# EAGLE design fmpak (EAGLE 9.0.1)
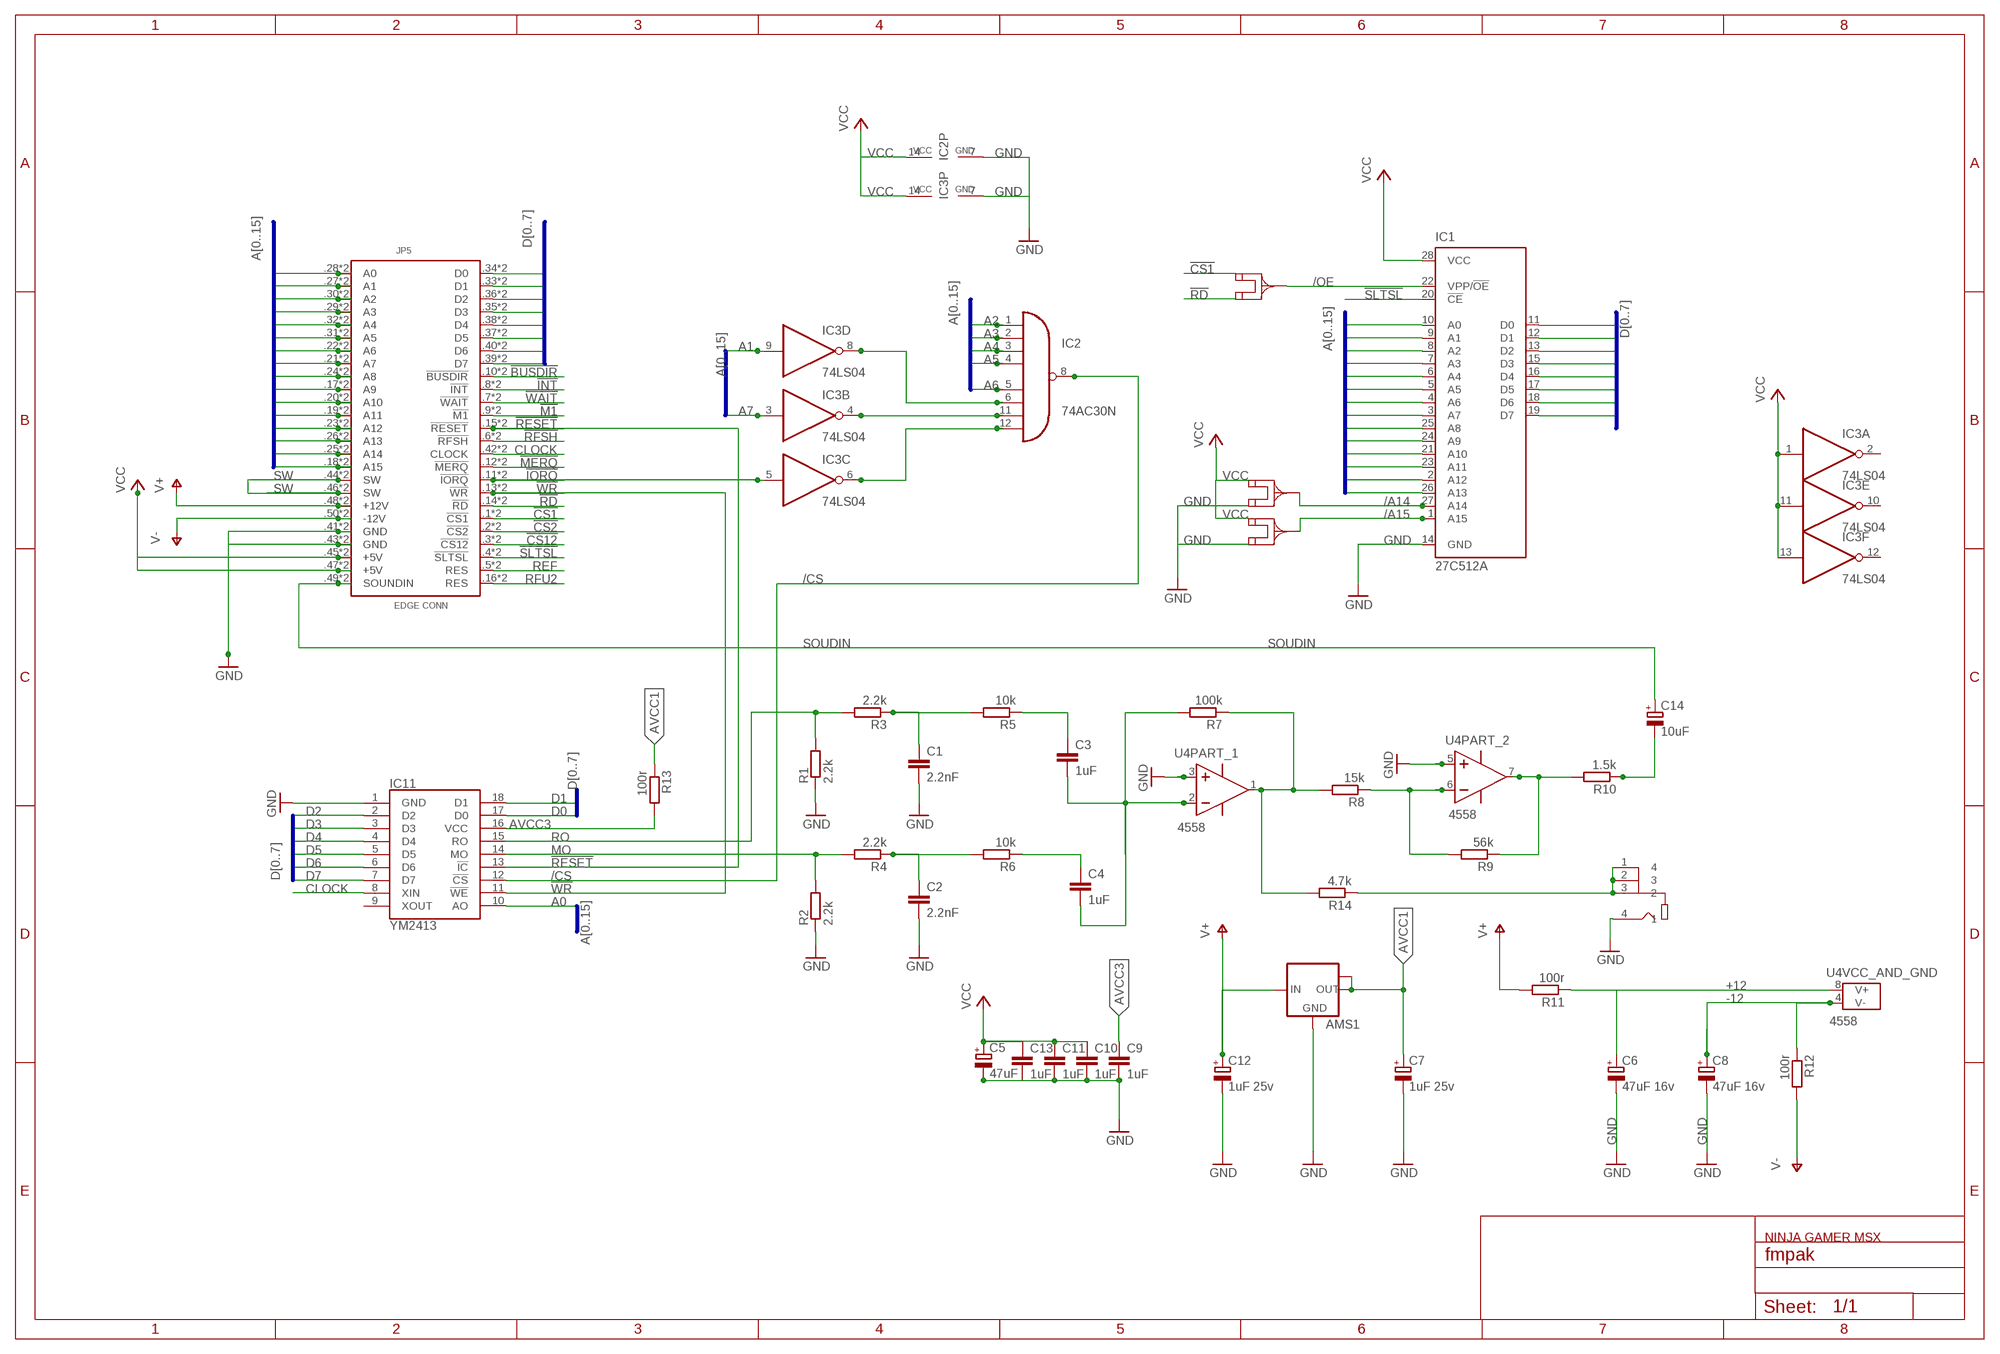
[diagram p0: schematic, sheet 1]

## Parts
AMS1  LM1117IMPX-5.0  [SOT223]
C1  2.2nF  C-EUC0805  [C0805]
C2  2.2nF  C-EUC0805  [C0805]
C3  1uF  C-EUC0805  [C0805]
C4  1uF  C-EUC0805  [C0805]
C5  47uF  CPOL-EUSMCC  [SMC_C]
C6  47uF 16v  CPOL-EUSMCC  [SMC_C]
C7  1uF 25v  CPOL-EUSMCB  [SMC_B]
C8  47uF 16v  CPOL-EUSMCC  [SMC_C]
C9  1uF  C-EUC0805  [C0805]
C10  1uF  C-EUC0805  [C0805]
C11  1uF  C-EUC0805  [C0805]
C12  1uF 25v  CPOL-EUSMCB  [SMC_B]
C13  1uF  C-EUC0805  [C0805]
C14  10uF  CPOL-EUSMCB  [SMC_B]
IC1  27C512A  27C512AP  [DIL28-6]
IC2  74AC30N  [DIL14]
IC3  74LS04  74LS04D  [SO14]
IC11  YM2413  [DIP762W56P254L2300H450Q18N]
J1  RCJ-04X  [CUI_RCJ-041]
JP5  MSXCART1  [MSXCART]
R1  2.2k  R-EU_R0805  [R0805]
R2  2.2k  R-EU_R0805  [R0805]
R3  2.2k  R-EU_R0805  [R0805]
R4  2.2k  R-EU_R0805  [R0805]
R5  10k  R-EU_R0805  [R0805]
R6  10k  R-EU_R0805  [R0805]
R7  100k  R-EU_R0805  [R0805]
R8  15k  R-EU_R0805  [R0805]
R9  56k  R-EU_R0805  [R0805]
R10  1.5k  R-EU_R0805  [R0805]
R11  100r  R-EU_R0805  [R0805]
R12  100r  R-EU_R0805  [R0805]
R13  100r  R-EU_R0805  [R0805]
R14  4.7k  R-EU_R0805  [R0805]
U4  4558  4558SO8  [SOP8]
U$1  JUMP-SMD  [A0R-JMP]
U$2  JUMP-SMD  [A0R-JMP]
U$3  JUMP-SMD  [A0R-JMP]

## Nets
!BUSDIR: JP5.9(!BUSDIR) JP5..10(!BUSDIR)
!CS1: JP5.1(!CS1) JP5..1(!CS1) U$2.1
!CS2: JP5.2(!CS2) JP5..2(!CS2)
!CS12: JP5.3(!CS12) JP5..3(!CS12)
!INT: JP5.8(!INT) JP5..8(!INT)
!IORQ: IC3.5(C:I) JP5.12(!IORQ) JP5..11(!IORQ)
!M1: JP5.10(!M1) JP5..9(!M1)
!MERQ: JP5.11(!MERQ) JP5..12(!MERQ)
!RD: JP5.14(!RD) JP5..14(!RD) U$2.3
!RESET: IC11.13(!IC) JP5.15(!RESET) JP5..15(!RESET)
!RFSH: JP5.6(!RFSH) JP5..6(!RFSH)
!SLTSL: IC1.20(!CE) JP5.4(!SLTSL) JP5..4(!SLTSL)
!WAIT: JP5.7(!WAIT) JP5..7(!WAIT)
!WR: IC11.11(!WE) JP5.13(!WR) JP5..13(!WR)
+12: C6.+ R11.1 U4.8(VCC_AND_GND:V+)
-12: C8.+ R12.1 U4.4(VCC_AND_GND:V-)
/A14: IC1.27(A14) U$1.2
/A15: IC1.1(A15) U$3.2
/CS: IC2.8(O) IC11.12(!CS)
/OE: IC1.22(VPP/!OE) U$2.2
A0: IC1.10(A0) IC11.10(AO) JP5.28(A0) JP5..28(A0)
A1: IC1.9(A1) IC3.9(D:I) JP5.27(A1) JP5..27(A1)
A2: IC1.8(A2) IC2.1(I0) JP5.30(A2) JP5..30(A2)
A3: IC1.7(A3) IC2.2(I1) JP5.29(A3) JP5..29(A3)
A4: IC1.6(A4) IC2.3(I2) JP5.32(A4) JP5..32(A4)
A5: IC1.5(A5) IC2.4(I3) JP5.31(A5) JP5..31(A5)
A6: IC1.4(A6) IC2.5(I4) JP5.22(A6) JP5..22(A6)
A7: IC1.3(A7) IC3.3(B:I) JP5.21(A7) JP5..21(A7)
A8: IC1.25(A8) JP5.24(A8) JP5..24(A8)
A9: IC1.24(A9) JP5.17(A9) JP5..17(A9)
A10: IC1.21(A10) JP5.20(A10) JP5..20(A10)
A11: IC1.23(A11) JP5.19(A11) JP5..19(A11)
A12: IC1.2(A12) JP5.23(A12) JP5..23(A12)
A13: IC1.26(A13) JP5.26(A13) JP5..26(A13)
A14: JP5.25(A14) JP5..25(A14)
A15: JP5.18(A15) JP5..18(A15)
AVCC1 [vcc]: AMS1.2(OUT) AMS1.TAB(OUT1) C7.+ R13.1
AVCC3: C9.1 IC11.16(VCC) R13.2
CLOCK: IC11.8(XIN) JP5.42(CLOCK) JP5..42(CLOCK)
D0: IC1.11(D0) IC11.17(D0) JP5.34(D0) JP5..34(D0)
D1: IC1.12(D1) IC11.18(D1) JP5.33(D1) JP5..33(D1)
D2: IC1.13(D2) IC11.2(D2) JP5.36(D2) JP5..36(D2)
D3: IC1.15(D3) IC11.3(D3) JP5.35(D3) JP5..35(D3)
D4: IC1.16(D4) IC11.4(D4) JP5.38(D4) JP5..38(D4)
D5: IC1.17(D5) IC11.5(D5) JP5.37(D5) JP5..37(D5)
D6: IC1.18(D6) IC11.6(D6) JP5.40(D6) JP5..40(D6)
D7: IC1.19(D7) IC11.7(D7) JP5.39(D7) JP5..39(D7)
GND: AMS1.1(GND) C1.2 C2.2 C5.- C6.- C7.- C8.- C9.2 C10.2 C11.2 C12.- C13.2 IC1.14(GND) IC2.7(GND) IC3.7(P:GND) IC11.1(GND) J1.4 JP5.41(GND) JP5.43(GND) JP5..41(GND) JP5..43(GND) R1.1 R2.1 U4.3(PART_1:IN+) U4.5(PART_2:IN+) U$1.3 U$3.3
MO: IC11.14(MO) R2.2 R4.2
N$2: C1.1 R3.1 R5.2
N$3: C3.1 R5.1
N$5: C2.1 R4.1 R6.2
N$6: C4.1 R6.1
N$7: C3.2 C4.2 R7.2 U4.2(PART_1:IN-)
N$8: R7.1 R8.2 R14.2 U4.1(PART_1:OUT)
N$9: R8.1 R9.2 U4.6(PART_2:IN-)
N$10: R9.1 R10.2 U4.7(PART_2:OUT)
N$11: C14.- R10.1
N$12: IC2.6(I5) IC3.8(D:O)
N$13: IC2.11(I6) IC3.4(B:O)
N$14: IC2.12(I7) IC3.6(C:O)
N$16: J1.1 J1.2 J1.3 R14.1
REF: JP5.5(RES) JP5..5(RES)
RFU2: JP5.16(RES) JP5..16(RES)
RO: IC11.15(RO) R1.2 R3.2
SOUDIN: C14.+ JP5.49(SOUNDIN) JP5..49(SOUNDIN)
SW: JP5.44(SW) JP5.46(SW) JP5..44(SW) JP5..46(SW)
V+: AMS1.3(IN) C12.+ JP5.48(+12V) JP5..48(+12V) R11.2
V-: JP5.50(-12V) JP5..50(-12V) R12.2
VCC: C5.+ C10.1 C11.1 C13.1 IC1.28(VCC) IC2.14(VCC) IC3.1(A:I) IC3.11(E:I) IC3.13(F:I) IC3.14(P:VCC) JP5.45(+5V) JP5.47(+5V) JP5..45(+5V) JP5..47(+5V) U$1.1 U$3.1
Unconnected: IC3.2(A:O) IC3.10(E:O) IC3.12(F:O) IC11.9(XOUT)

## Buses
D[0..7]
A[0..15]

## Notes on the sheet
- NINJA GAMER MSX

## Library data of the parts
AMS1 = lm1117:LM1117IMPX-*
C1-C4 C9-C11 C13 = rcl:C-EU: CAPACITOR, European symbol
C5-C8 C12 C14 = rcl:CPOL-EU: POLARIZED CAPACITOR, European symbol
IC1 = microchip:27*512A: CMOS EPROM 512 K (64 K x 8); MPN: M27C512-90B6; OC_FARNELL: 1642690; OC_NEWARK: 20M6389
IC2 = 74xx-eu:74*30: 8-input NAND gate
IC3 = 74xx-eu:74*04: Hex INVERTER
IC11 = YM2413:YM2413: SOUND GENERATOR CIRCUIT, 18 Pin, DIP Source: Datasheet; DESCRIPTION: SOUND GENERATOR CIRCUIT, 18 Pin, DIP; HEIGHT: 4.5mm; MANUFACTURER_NAME: Yamaha; MANUFACTURER_PART_NUMBER: YM2413
J1 = RCA-JACK:RCJ-04X: 1 Port, Right Angle, Through Hole, RCA Jack Connector; MF: CUI Inc; MP: RCJ-041; PACKAGE: N/A; STANDARD: Manufacturer recommendations
JP5 = msx-con:MSXCART
R1-R14 = rcl:R-EU_: RESISTOR, European symbol
U4 = common:4558
U$1-U$3 = jump-PERSONALIZADO 3 PAD:JUMP-SMD

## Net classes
0 default: width 0.254 mm
1 vcc: width 0.305 mm
2 gnd: width 0.305 mm

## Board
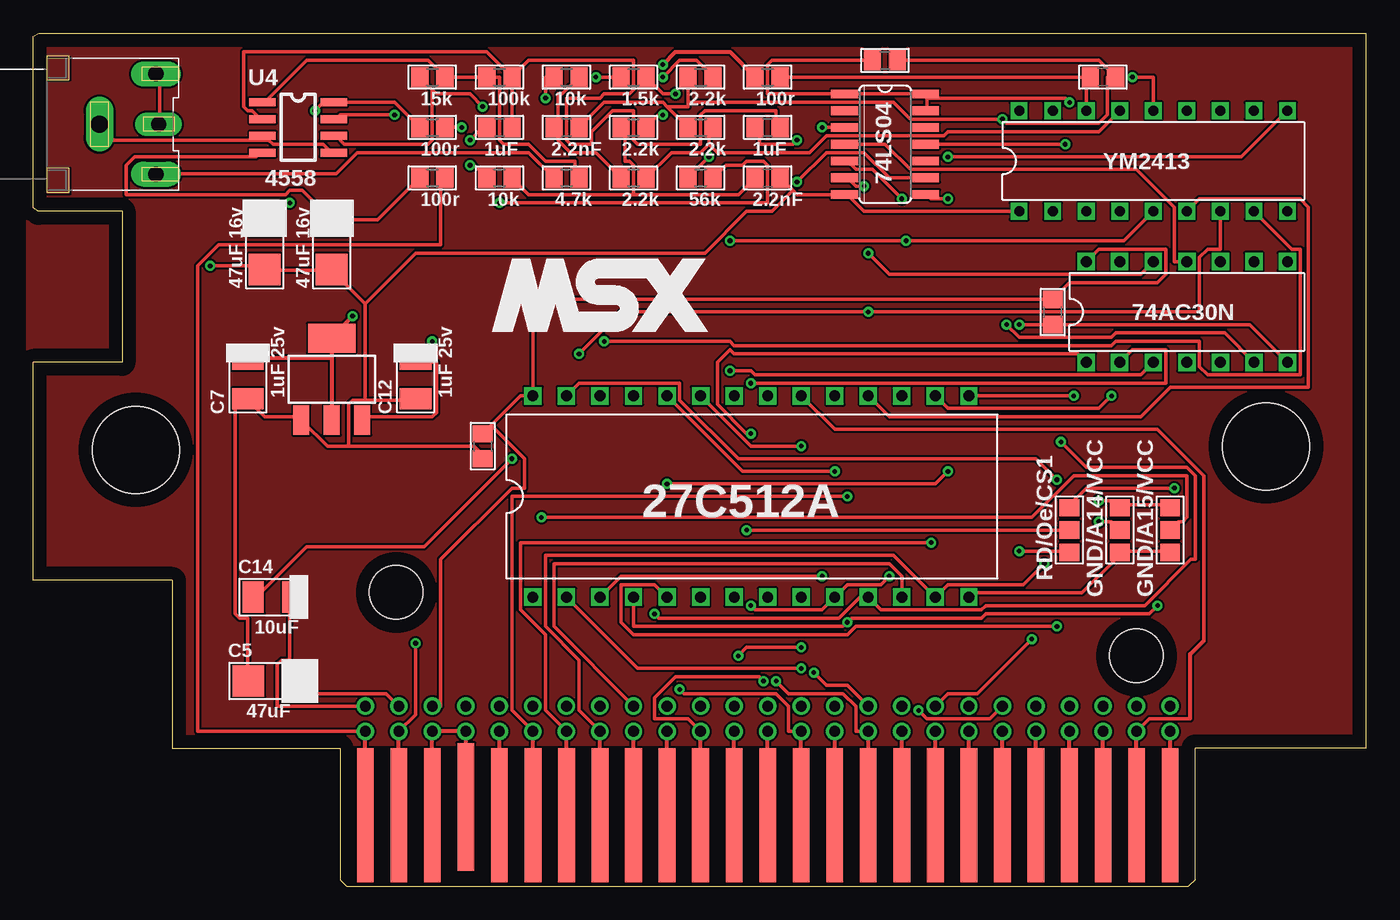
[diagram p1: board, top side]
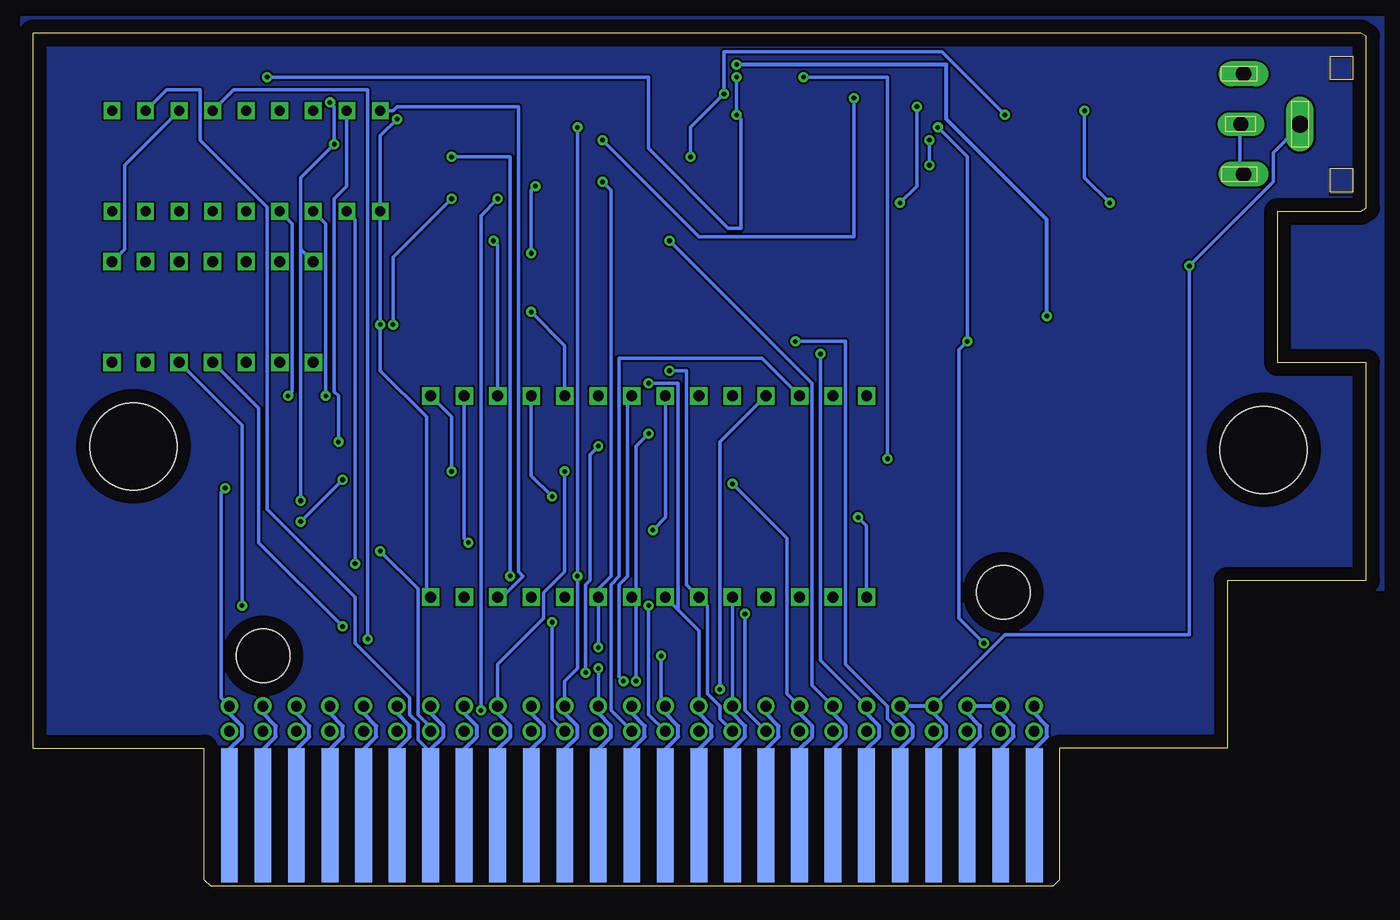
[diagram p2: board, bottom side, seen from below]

Size 101 x 64.62 mm. Coordinates in mm from the lower left corner, seen from the top.
Copper layers (1*16): Top 0.035mm / dielectric 1.5mm / Bottom 0.035mm
Design rules "default *": minimum track width 6mil, minimum drill 0.35mm, track to track 6mil, track to pad 6mil, pad to pad 6mil, via to via 6mil, smd to smd 6mil, copper to edge 40mil, drill to drill 6mil, minimum pad ring 10mil, minimum via ring 8mil, stop-mask expansion 0mil, vias tented up to drill 20mil, thermal gap 10mil

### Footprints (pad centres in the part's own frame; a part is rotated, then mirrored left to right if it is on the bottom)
SOT223 = smd 1.219 x 2.235: 1 -2.311,-3.099; 2 0,-3.099; 3 2.311,-3.099 | smd 3.6 x 2.2: TAB 0,3.099
C0805 = smd 1.3 x 1.5: 1 -0.95,0; 2 0.95,0
SMC_C = smd 2.4 x 2.4: + 1.865,0; - -1.865,0
SMC_B = smd 1.6 x 2.4: + 1.5,0; - -1.5,0
DIL28-6 = drill 0.813 square: 1 -16.51,-7.62; 2 -13.97,-7.62; 3 -11.43,-7.62; 4 -8.89,-7.62; 5 -6.35,-7.62; 6 -3.81,-7.62; 7 -1.27,-7.62; 8 1.27,-7.62; 9 3.81,-7.62; 10 6.35,-7.62; 11 8.89,-7.62; 12 11.43,-7.62; 13 13.97,-7.62; 14 16.51,-7.62; 15 16.51,7.62; 16 13.97,7.62; 17 11.43,7.62; 18 8.89,7.62; 19 6.35,7.62; 20 3.81,7.62; 21 1.27,7.62; 22 -1.27,7.62; 23 -3.81,7.62; 24 -6.35,7.62; 25 -8.89,7.62; 26 -11.43,7.62; 27 -13.97,7.62; 28 -16.51,7.62
DIL14 = drill 0.813 square: 1 -7.62,-3.81; 2 -5.08,-3.81; 3 -2.54,-3.81; 4 0,-3.81; 5 2.54,-3.81; 6 5.08,-3.81; 7 7.62,-3.81; 8 7.62,3.81; 9 5.08,3.81; 10 2.54,3.81; 11 0,3.81; 12 -2.54,3.81; 13 -5.08,3.81; 14 -7.62,3.81
SO14 = smd 0.66 x 2.032: 1 -3.81,-3.073; 2 -2.54,-3.073; 3 -1.27,-3.073; 4 0,-3.073; 5 1.27,-3.073; 6 2.54,-3.073; 7 3.81,-3.073; 8 3.81,3.073; 9 2.54,3.073; 10 1.27,3.073; 11 0,3.073; 12 -1.27,3.073; 13 -2.54,3.073; 14 -3.81,3.073
DIP762W56P254L2300H450Q18N = drill 0.76 pad 1.16 square: 1 -10.16,-3.81; 2 -7.62,-3.81; 3 -5.08,-3.81; 4 -2.54,-3.81; 5 0,-3.81; 6 2.54,-3.81; 7 5.08,-3.81; 8 7.62,-3.81; 9 10.16,-3.81; 10 10.16,3.81; 11 7.62,3.81; 12 5.08,3.81; 13 2.54,3.81; 14 0,3.81; 15 -2.54,3.81; 16 -5.08,3.81; 17 -7.62,3.81; 18 -10.16,3.81
CUI_RCJ-041 = drill 1.143 pad 1.905 long: 1 -3.533,-8.275; 3 4.067,-8.275 | drill 1.143 pad 1.778 long: 2 0.257,-8.481 | drill 1.3 pad 2.1 long: 4 0.254,-4
MSXCART = drill 0.813 pad 1.143: 1 30.48,14.605; 2 30.48,12.7; 3 27.94,14.605; 4 27.94,12.7; 5 25.4,14.605; 6 25.4,12.7; 7 22.86,14.605; 8 22.86,12.7; 9 20.32,12.7; 10 20.32,14.605; 11 17.78,12.7; 12 17.78,14.605; 13 15.24,14.605; 14 15.24,12.7; 15 12.7,14.605; 16 12.7,12.7; 17 10.16,14.605; 18 10.16,12.7; 19 7.62,14.605; 20 7.62,12.7; 21 5.08,14.605; 22 5.08,12.7; 23 2.54,14.605; 24 2.54,12.7; 25 0,14.605; 26 0,12.7; 27 -2.54,14.605; 28 -2.54,12.7; 29 -5.08,14.605; 30 -5.08,12.7; 31 -7.62,14.605; 32 -7.62,12.7; 33 -10.16,14.605; 34 -10.16,12.7; 35 -12.7,14.605; 36 -12.7,12.7; 37 -15.24,14.605; 38 -15.24,12.7; 39 -17.78,14.605; 40 -17.78,12.7; 41 -20.32,14.605; 42 -20.32,12.7; 43 -22.86,14.605; 44 -22.86,12.7; 45 -25.4,14.605; 46 -25.4,12.7; 47 -27.94,14.605; 48 -27.94,12.7; 49 -30.48,14.605; 50 -30.48,12.7 | smd 1.27 x 10.16 bottom: .1 30.48,6.35; .3 27.94,6.35; .5 25.4,6.35; .7 22.86,6.35; .9 20.32,6.35; .11 17.78,6.35; .13 15.24,6.35; .15 12.7,6.35; .17 10.16,6.35; .19 7.62,6.35; .21 5.08,6.35; .23 2.54,6.35; .25 0,6.35; .27 -2.54,6.35; .29 -5.08,6.35; .31 -7.62,6.35; .33 -10.16,6.35; .35 -12.7,6.35; .37 -15.24,6.35; .39 -17.78,6.35; .41 -20.32,6.35; .43 -22.86,6.35; .45 -25.4,6.35; .47 -27.94,6.35; .49 -30.48,6.35 | smd 1.27 x 10.16: .2 30.48,6.35; .4 27.94,6.35; .6 25.4,6.35; .8 22.86,6.35; .10 20.32,6.35; .12 17.78,6.35; .14 15.24,6.35; .16 12.7,6.35; .18 10.16,6.35; .20 7.62,6.35; .22 5.08,6.35; .24 2.54,6.35; .26 0,6.35; .28 -2.54,6.35; .30 -5.08,6.35; .32 -7.62,6.35; .34 -10.16,6.35; .36 -12.7,6.35; .38 -15.24,6.35; .40 -17.78,6.35; .42 -20.32,6.35; .46 -25.4,6.35; .48 -27.94,6.35; .50 -30.48,6.35 | smd 1.27 x 9.652: .44 -22.86,6.985 | hole 4.064: -28.14,23.215; 27.929,18.415 | hole 6.604: 37.748,34.277; -47.859,34.007
R0805 = smd 1.3 x 1.5: 1 -0.95,0; 2 0.95,0
SOP8 = smd 2 x 0.6: 1 -2.7,1.905; 2 -2.7,0.635; 3 -2.7,-0.635; 4 -2.7,-1.905; 5 2.7,-1.905; 6 2.7,-0.635; 7 2.7,0.635; 8 2.7,1.905
A0R-JMP = smd 1.5 x 1.3: 1 0,1.7; 2 0,0; 3 0,-1.7

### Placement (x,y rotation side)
AMS1  22.62,38.42 0 top
C1  40.41,57.47 0 top
C2  55.64,53.66 0 top
C3  55.64,57.47 0 top
C4  35.33,57.47 0 top
C5  18.18,15.56 0 top
C6  17.55,48.58 90 top
C7  16.27,38.42 90 top
C8  22.62,48.58 90 top
C9  81.04,61.28 0 top
C10  64.53,62.55 0 top
C11  34.05,33.34 270 top
C12  28.97,38.42 90 top
C13  77.23,43.5 270 top
C14  18.18,21.91 0 top
IC1  54.38,29.53 0 top
IC2  87.39,43.5 0 top
IC3  64.53,56.2 270 top
IC11  84.85,54.93 0 top
J1  1.03,57.47 90 top
JP5  55.64,-0.95 0 top
R1  50.56,57.47 0 top
R2  50.56,61.28 0 top
R3  45.48,53.66 0 top
R4  45.48,57.47 0 top
R5  40.41,61.28 0 top
R6  35.33,53.66 0 top
R7  35.33,61.28 0 top
R8  30.25,61.28 0 top
R9  50.56,53.66 0 top
R10  45.48,61.28 0 top
R11  30.25,57.47 0 top
R12  30.25,53.66 0 top
R13  55.64,61.28 0 top
R14  40.41,53.66 0 top
U4  20.08,57.47 0 top
U$1  82.31,26.99 0 top
U$2  78.5,26.99 0 top
U$3  86.12,26.99 0 top

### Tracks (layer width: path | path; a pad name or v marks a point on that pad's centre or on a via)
!BUSDIR
  Top 0.305: JP5..10 JP5.9
!CS1  (via drill 0.35)
  Top 0.254: v86.44,30.16 79.78,30.16 78.5,28.89 U$2.1
  Bottom 0.254: v86.44,30.16 86.76,29.85 86.76,14.29 JP5.1
  Bottom 0.305: JP5..1 86.12,10.38 85.16,11.35 85.16,12.15 86.12,13.11 JP5.1
!CS2
  Top 0.305: JP5..2 JP5.2
!CS12
  Bottom 0.305: JP5..3 83.58,10.38 82.62,11.35 82.62,12.15 83.58,13.11 JP5.3
!INT
  Top 0.305: JP5..8 JP5.8
!IORQ  (via drill 0.35)
  Top 0.254: v65.81,52.07 63.58,54.29 62.31,54.29 61.68,54.93 IC3.5 | v67.07,13.33 67.71,12.7 72.47,12.7 JP5.12
  Bottom 0.254: v65.81,52.07 67.07,50.8 v67.07,13.33
  Bottom 0.305: JP5..11 73.42,10.38 72.46,11.35 72.46,12.15 73.42,13.11 JP5.12
!M1
  Bottom 0.305: JP5..9 75.97,10.38 75,11.35 75,12.15 75.97,13.11 JP5.10
!MERQ
  Top 0.305: JP5..12 JP5.11
!RD  (via drill 0.35)
  Top 0.254: v74.69,25.4 78.5,25.4 U$2.3
  Top 0.305: JP5..14 JP5.14
  Bottom 0.254: v74.69,25.4 71.84,22.54 71.84,13.02 70.88,12.06 JP5.14
!RESET  (via drill 0.35)
  Top 0.254: v75.65,18.73 71.52,14.61 69.3,14.61 JP5.15
  Bottom 0.254: IC11.13 85.81,60.32 75.65,60.32 v75.65,18.73
  Bottom 0.305: JP5..15 68.34,10.38 67.38,11.35 67.38,12.15 68.34,13.11 JP5.15
!RFSH
  Top 0.305: JP5..6 JP5.6
!SLTSL
  Top 0.254: IC1.20 60.72,34.61 85.17,34.61 88.66,31.11 88.66,18.61 | 87.65,12.7 84.54,12.7 JP5.4
  Top 0.305: JP5..4 JP5.4 | 87.65,12.7 87.65,17.59 88.66,18.61
!WAIT
  Bottom 0.305: JP5..7 78.5,10.38 77.54,11.35 77.54,12.15 78.5,13.11 JP5.7
!WR
  Bottom 0.254: IC11.11 90.89,60.32 88.35,60.32 88.35,56.51 83.27,51.43 83.27,28.57 76.6,21.91 76.6,18.41 72.47,14.29 72.47,13.02 71.84,12.38 71.84,11.11 70.88,10.16
  Bottom 0.305: JP5..13 70.88,10.16 70.88,10.38 69.92,11.35 69.92,12.15 70.88,13.11 JP5.13
+12  (via drill 0.35)
  Top 0.254: R11.1 27.39,59.37 U4.8 21.99,59.37 v21.36,58.74 | v19.45,51.75 18.81,51.75 17.55,50.48 C6.+
  Bottom 0.254: v19.45,51.75 21.36,53.66 v21.36,58.74
-12
  Top 0.254: 22.62,50.48 26.12,50.48 R12.1 | 22.62,50.48 20.4,52.71 19.45,52.71 19.13,52.39 7.07,52.39 7.07,54.61 7.7,55.25 16.91,55.25 17.23,55.56 U4.4 | 22.62,50.48 C8.+
/A14  (via drill 0.35)
  Top 0.254: U$1.2 81.68,27.62 v80.73,27.62 | v77.55,30.8 75.97,32.39 53.42,32.39 48.98,36.83 48.98,38.1 41.36,38.1 IC1.27
  Bottom 0.254: v77.55,30.8 v80.73,27.62
/A15  (via drill 0.35)
  Top 0.254: U$3.2 86.76,27.62 87.08,27.62 87.39,27.94 87.39,31.11 78.82,31.11 75.65,27.94 v38.5,27.94
  Bottom 0.254: v38.5,27.94 37.86,27.3 IC1.1
/CS
  Bottom 0.254: IC11.12 94.06,54.61 94.06,48.26 IC2.8
/OE  (via drill 0.35)
  Top 0.254: v54.06,26.99 U$2.2
  Bottom 0.254: v54.06,26.99 53.1,27.94 IC1.22
A0  (via drill 0.35)
  Top 0.254: IC11.10 91.52,55.25 v69.3,55.25 | v64.85,23.5 64.22,22.86 61.68,22.86 IC1.10 59.77,20.95 54.69,20.95 v54.38,21.27
  Top 0.305: JP5..28 JP5.28
  Bottom 0.254: v69.3,55.25 64.85,55.25 v64.85,23.5 | JP5.28 54.38,13.02 v54.38,21.27
A1  (via drill 0.35)
  Top 0.254: IC3.9 64.85,53.66 62.95,55.56 60.09,55.56 v57.87,53.34 | v53.42,17.46 54.06,18.1 v58.18,18.1
  Bottom 0.254: v57.87,53.34 57.23,52.71 57.23,23.5 58.18,22.54 IC1.9 v58.18,18.1 | JP5.27 53.42,13.97 v53.42,17.46
  Bottom 0.305: JP5..27 53.1,10.38 52.14,11.35 52.14,12.15 53.1,13.11 JP5.27
A2  (via drill 0.35)
  Top 0.254: v55.33,15.56 55.01,15.88 48.66,15.88 47.07,14.29 47.07,12.7 49.61,12.7 JP5.30 | IC2.1 79.14,40.32 53.1,40.32 52.79,40.64 51.84,39.69 51.84,36.51 54.06,34.29 v54.38,34.29
  Top 0.305: JP5..30 JP5.30
  Bottom 0.254: v55.33,15.56 55.33,21.59 | v54.38,34.29 55.33,33.34 55.33,21.59 | 55.33,21.59 IC1.8
A3  (via drill 0.35)
  Top 0.254: IC2.2 83.27,40.64 85.81,40.64 85.81,38.1 v54.38,38.1
  Bottom 0.254: 52.15,20.95 50.56,19.37 JP5.29 | 52.15,20.95 IC1.7 | v54.38,38.1 52.15,38.1 52.15,20.95
  Bottom 0.305: JP5..29 50.56,10.38 49.6,11.35 49.6,12.15 50.56,13.11 JP5.29
A4  (via drill 0.35)
  Top 0.254: IC2.3 83.9,38.74 54.69,38.74 54.38,39.05 v52.79,39.05
  Top 0.305: JP5..32 JP5.32
  Bottom 0.254: JP5.32 48.98,12.7 48.98,13.65 49.93,14.61 49.93,21.27 IC1.6 51.52,22.86 51.52,39.05 v52.79,39.05
A5  (via drill 0.35)
  Top 0.254: v77.55,19.68 62.31,19.68 61.68,19.05 45.48,19.05 44.53,20 44.53,22.86 47.07,22.86 IC1.5
  Bottom 0.254: JP5.31 IC1.5 | IC2.4 83.9,36.19 83.9,26.04 v77.55,19.68
  Bottom 0.305: JP5..31 48.02,10.38 47.06,11.35 47.06,12.15 48.02,13.11 JP5.31
A6  (via drill 0.35)
  Top 0.254: IC1.4 45.48,19.68 61.36,19.68 v61.68,20 61.99,20.32 71.84,20.32 72.16,20.64 84.54,20.64 v85.17,21.27
  Top 0.305: JP5..22 JP5.22
  Bottom 0.254: v61.68,20 61.68,12.7 JP5.22 | IC2.5 85.17,34.93 v85.17,21.27
A7  (via drill 0.35)
  Top 0.254: v59.77,57.47 IC3.3 | IC1.3 44.53,23.5 v59.77,23.5
  Bottom 0.254: v59.77,57.47 v59.77,23.5 59.77,16.51 60.72,15.56 JP5.21
  Bottom 0.305: JP5..21 60.72,10.38 59.76,11.35 59.76,12.15 60.72,13.11 JP5.21
A8  (via drill 0.35)
  Top 0.254: v48.98,14.92 49.3,14.61 56.28,14.61 57.23,13.65 57.23,11.75 JP5.24
  Top 0.305: JP5..24 JP5.24
  Bottom 0.254: IC1.25 48.98,33.65 v48.98,14.92
A9  (via drill 0.35)
  Top 0.254: IC1.24 53.74,31.43 v60.72,31.43
  Bottom 0.254: v60.72,31.43 60.72,23.81 62.31,22.23 62.31,20.32 65.81,16.83 JP5.17
  Bottom 0.305: JP5..17 65.81,10.38 64.84,11.35 64.84,12.15 65.81,13.11 JP5.17
A10  (via drill 0.35)
  Top 0.254: v56.28,15.56 57.23,14.61 61.36,14.61 62.31,13.65 62.31,11.75 JP5.20
  Top 0.305: JP5..20 JP5.20
  Bottom 0.254: IC1.21 55.96,36.83 55.96,23.5 56.6,22.86 56.6,15.88 v56.28,15.56
A11  (via drill 0.35)
  Top 0.254: IC1.23 54.38,33.34 v58.18,33.34 | v59.14,16.19 60.09,15.24 61.68,15.24 JP5.19
  Bottom 0.254: v58.18,33.34 58.82,32.7 58.82,23.18 59.14,22.86 v59.14,16.19
  Bottom 0.305: JP5..19 63.27,10.38 62.3,11.35 62.3,12.15 63.27,13.11 JP5.19
A12  (via drill 0.35)
  Top 0.254: IC1.2 45.8,16.51 v58.18,16.51
  Bottom 0.254: JP5.23 v58.18,16.51
  Bottom 0.305: JP5..23 58.18,10.38 57.22,11.35 57.22,12.15 58.18,13.11 JP5.23
A13
  Top 0.305: JP5..26 JP5.26
  Bottom 0.254: IC1.26 45.8,40 56.6,40 56.6,23.5 57.23,22.86 57.23,13.33 JP5.26
A14
  Bottom 0.305: JP5..25 55.64,10.38 54.68,11.35 54.68,12.15 55.64,13.11 JP5.25
A15
  Top 0.305: JP5..18 JP5.18
AVCC1  (via drill 0.35)
  Top 0.305: v47.71,62.23 48.66,63.18 52.79,63.18 R13.1 | v24.21,43.18 22.62,41.59 AMS1.TAB 22.62,40 | 22.62,40 AMS1.2 | 22.62,40 16.27,40 C7.+
  Bottom 0.305: v47.71,62.23 31.83,62.23 31.83,58.1 24.21,50.48 v24.21,43.18
AVCC3
  Top 0.254: 79.78,61.28 C9.1 | 79.78,61.28 R13.2 | 79.78,61.28 IC11.16
CLOCK  (via drill 0.35)
  Top 0.254: IC11.8 95.33,48.26 95.97,48.26 95.97,38.74 88.98,38.74 88.35,39.37 88.35,41.28 82,41.28 81.68,40.96 53.1,40.96 52.79,41.28 v43.26,41.28
  Top 0.305: JP5..42 JP5.42
  Bottom 0.254: v43.26,41.28 39.45,41.28 39.45,16.83 36.28,13.65 36.28,12.7 JP5.42
D0  (via drill 0.35)
  Top 0.254: v77.87,33.65 79.78,31.75 87.39,31.75 88.03,31.11 88.03,24.77 87.71,24.77 84.22,21.27 72.16,21.27 71.84,20.95 64.22,20.95 IC1.11 62.63,21.91 61.04,20.32 47.39,20.32 v47.07,20.64
  Top 0.305: JP5..34 JP5.34
  Bottom 0.254: IC11.17 77.23,53.02 78.19,52.07 78.19,37.47 77.87,37.15 v77.87,33.65 | JP5.34 47.07,13.33 v47.07,20.64
D1
  Top 0.254: JP5.33 39.45,19.68 39.45,24.45 64.85,24.45 65.81,23.5 IC1.12
  Bottom 0.254: IC11.18 73.74,58.74 73.42,59.06 64.22,59.06 64.22,23.81 63.9,23.5 65.49,21.91 IC1.12
  Bottom 0.305: JP5..33 45.48,10.38 44.52,11.35 44.52,12.15 45.48,13.11 JP5.33
D2  (via drill 0.35)
  Top 0.254: v76.6,24.45 75.01,22.86 69.3,22.86 IC1.13 65.17,25.08 38.82,25.08 38.82,19.68 41.36,17.14 41.36,13.33 JP5.36
  Top 0.305: JP5..36 JP5.36
  Bottom 0.254: IC11.2 76.6,50.48 v76.6,24.45
D3  (via drill 0.35)
  Top 0.254: IC1.15 v78.82,37.15 | v69.3,31.43 68.34,30.48 v48.02,30.48
  Bottom 0.254: IC11.3 78.82,50.17 v78.82,37.15 | IC1.15 69.3,35.56 v69.3,31.43 | v48.02,30.48 43.9,26.35 43.9,14.61 JP5.35
  Bottom 0.305: JP5..35 42.94,10.38 41.98,11.35 41.98,12.15 42.94,13.11 JP5.35
D4  (via drill 0.35)
  Top 0.254: v81.68,37.15 80.73,36.19 69.3,36.19 IC1.16 | JP5.38 38.82,13.33 38.82,19.05 36.91,20.95 36.91,26.04 v68.03,26.04
  Top 0.305: JP5..38 JP5.38
  Bottom 0.254: IC11.4 81.36,50.17 81.36,37.47 v81.68,37.15 | v68.03,26.04 68.34,26.35 IC1.16
D5  (via drill 0.35)
  Top 0.254: IC11.5 82.63,48.89 v66.12,48.89 v52.79,48.89
  Bottom 0.254: v66.12,48.89 65.81,48.58 IC1.17 | JP5.37 41.99,15.24 41.99,38.1 v52.79,48.89
  Bottom 0.305: JP5..37 40.41,10.38 39.44,11.35 39.44,12.15 40.41,13.11 JP5.37
D6  (via drill 0.35)
  Top 0.254: IC11.6 88.35,52.07 95.97,52.07 96.6,51.43 96.6,37.78 86.12,37.78 83.9,35.56 64.85,35.56 IC1.18 | JP5.40 36.28,13.33 36.28,29.53 v61.68,29.53
  Top 0.305: JP5..40 JP5.40
  Bottom 0.254: v61.68,29.53 63.27,31.11 IC1.18
D7  (via drill 0.35)
  Top 0.254: IC11.7 89.94,48.26 88.98,48.26 88.35,47.62 88.35,43.5 v63.27,43.5 44.53,43.5 v41.36,40.32
  Bottom 0.254: v63.27,43.5 60.72,40.96 IC1.19 | JP5.39 41.36,17.14 v41.36,40.32
  Bottom 0.305: JP5..39 37.86,10.38 36.9,11.35 36.9,12.15 37.86,13.11 JP5.39
GND  (via drill 0.35)
  Top 0.254: 17.86,56.51 17.55,56.83 U4.3 | 17.86,56.51 18.18,56.2 21.99,56.2 22.62,55.56 U4.5 | 17.86,56.51 6.11,56.51 5.16,57.47 J1.4 | 22.62,46.67 17.55,46.67 C6.- 17.55,46.99 v13.42,46.99 | 23.89,33.34 22.31,33.34 20.4,35.24 AMS1.1 20.08,35.56 17.55,35.56 16.27,36.83 | 23.89,33.34 33.42,33.34 34.05,32.7 C11.2 | 16.27,36.83 15.32,36.83 15.32,20.64 15.64,20.32 16.27,20.32 16.27,15.56 C5.- | 16.27,36.83 C7.- | 25.16,36.83 24.21,36.83 23.89,36.51 23.89,33.34 | 25.16,36.83 28.97,36.83 C12.- | 25.16,44.13 22.62,46.67 | 25.16,36.83 25.16,44.13 | 22.62,46.67 C8.- | 48.02,59.06 R1.1 | 48.02,59.06 47.71,59.37 43.26,59.37 C1.2 | 49.61,59.37 49.61,59.06 48.02,59.06 | 49.61,59.37 R2.1 | C10.2 80.73,62.55 C9.2 81.36,61.28 81.36,58.42 80.73,57.79 73.74,57.79 v73.42,58.1 66.44,58.1 65.17,59.37 49.61,59.37 | C13.2 92.16,42.54 IC2.7 | U$3.3 86.12,25.4 82.31,25.4 U$1.3 82.31,25.08 79.46,22.23 71.2,22.23 IC1.14 | 57.55,52.71 57.87,52.39 IC3.7 61.68,52.39 62.95,51.12 IC11.1 | 57.55,52.71 C2.2 | v74.69,42.54 C13.2 | C13.2 | 25.16,44.13 28.97,47.94 50.88,47.94 54.06,51.12 55.96,51.12 57.55,52.71
  Bottom 0.254: J1.4 5.16,57.47 7.07,55.56 7.07,53.34 v13.42,46.99 13.42,19.05 27.39,19.05 JP5.43 | IC1.14 71.2,22.23 71.2,35.56 74.69,39.05 v74.69,42.54 IC11.1 74.69,56.83 v73.42,58.1
  Bottom 0.305: JP5..41 35.33,10.38 34.36,11.35 34.36,12.15 35.33,13.11 35.33,13.53 | 35.33,13.53 JP5.41 | JP5..43 32.78,10.38 31.82,11.35 31.82,12.15 32.78,13.11 JP5.43 35.2,13.65 35.33,13.53
MO  (via drill 0.35)
  Top 0.254: v47.71,58.42 47.39,58.42 R4.2 | v47.71,61.28 48.98,62.55 50.25,62.55 R2.2 | IC11.14 84.85,61.28 v83.27,61.28
  Bottom 0.254: v47.71,61.28 v47.71,58.42 47.39,58.1 47.39,49.85 48.34,49.85 54.38,55.88 54.38,61.28 v83.27,61.28
N$1
  pour Top: 23.13,10.22 23.13,10.73 24.91,10.73 88.16,10.73 88.16,10.22 88.92,10.22 101.36,10.22 101.36,11.75 101.36,65.09 18.05,65.09 -0.49,65.09 -0.49,57.72 -0.49,22.92 10.18,22.92 10.18,10.22 17.55,10.22
N$2
  Top 0.254: 39.77,57.47 39.77,60.01 40.09,60.01 R5.2 | 39.77,57.47 39.77,56.51 40.72,55.56 42.63,55.56 R3.1 | 39.77,57.47 C1.1
N$3  (via drill 0.35)
  Top 0.254: v57.87,56.51 57.55,56.2 55.01,56.2 55.01,57.47 C3.1 | v38.82,59.69 38.82,61.28 R5.1
  Bottom 0.254: v57.87,56.51 50.56,49.21 38.82,49.21 v38.82,59.69
N$4
  pour Bottom: 23.13,9.97 23.13,10.73 23.89,10.73 88.16,10.73 88.16,9.97 89.94,9.97 101.87,9.97 101.87,10.99 101.87,65.85 5.35,65.85 -1.25,65.85 -1.25,63.31 -1.25,22.42 9.67,22.42 9.67,9.97
N$5
  Top 0.254: 45.48,52.39 53.42,52.39 C2.1 | 45.48,52.39 37.55,52.39 R6.2 | 45.48,52.39 45.48,54.61 45.17,54.93 44.85,54.93 44.85,57.47 R4.1
N$6  (via drill 0.35)
  Top 0.254: v33.1,54.61 33.42,54.61 R6.1 | v33.1,56.51 34.05,57.47 C4.1
  Bottom 0.254: v33.1,56.51 v33.1,54.61
N$7
  Top 0.254: R7.2 C4.2 | R7.2 37.55,62.55 45.48,62.55 45.48,60.32 45.17,60.01 43.26,60.01 42.94,59.69 40.41,59.69 40.41,56.51 40.72,56.2 42.31,56.2 42.31,57.15 43.9,58.74 45.48,58.74 45.48,56.51 45.8,56.2 50.56,56.2 50.56,58.42 50.88,58.74 56.28,58.74 56.28,57.47 C3.2 | R7.2 34.37,63.18 15.96,63.18 15.96,59.06 16.27,58.74 16.59,58.74 17.23,58.1 U4.2 | R7.2
N$8
  Top 0.254: R8.2 R7.1 35.33,61.28 35.33,56.51 35.64,56.2 37.55,56.2 38.82,54.93 41.04,54.93 41.04,53.66 R14.2 | R8.2 29.93,62.55 20.72,62.55 17.55,59.37 U4.1 | R8.2
N$9  (via drill 0.35)
  Top 0.254: v35.33,51.75 55.64,51.75 55.64,54.61 55.33,54.93 54.06,54.93 53.74,54.61 52.47,54.61 R9.2 | v34.05,59.06 33.1,60.01 30.56,60.01 30.25,60.32 | 30.25,60.32 R8.1 | 30.25,60.32 30.25,56.51 29.93,56.2 23.58,56.2 22.94,56.83 U4.6
  Bottom 0.254: v35.33,51.75 34.05,53.02 v34.05,59.06
N$10  (via drill 0.35)
  Top 0.254: v48.66,60.01 47.71,60.01 R10.2 | v51.2,55.25 R9.1 | v27.39,58.42 23.26,58.42 22.94,58.1 U4.7
  Bottom 0.254: v51.2,55.25 51.2,57.47 v48.66,60.01 48.66,63.18 32.15,63.18 v27.39,58.42
N$11  (via drill 0.35)
  Top 0.254: v42.63,61.28 R10.1 | v36.28,32.39 29.61,25.72 20.72,25.72 16.91,21.91 C14.-
  Bottom 0.254: v42.63,61.28 36.28,61.28 v36.28,32.39
N$12  (via drill 0.35)
  Top 0.254: v69.3,52.07 68.03,52.07 67.71,52.39 IC3.8 | v73.74,42.54 74.69,41.59 81.68,41.59 82,41.91 90.25,41.91 IC2.6
  Bottom 0.254: v69.3,52.07 73.74,47.62 v73.74,42.54
N$13
  Top 0.254: IC3.4 64.53,56.2 66.44,54.29 83.58,54.29 86.44,51.43 86.44,47.31 IC2.11
N$14  (via drill 0.35)
  Top 0.254: v62.95,53.02 62.31,53.02 61.68,53.66 IC3.6 | v63.27,47.94 64.85,46.36 83.9,46.36 IC2.12
  Bottom 0.254: v62.95,53.02 63.27,52.71 v63.27,47.94
N$16
  Top 0.254: J1.2 9.61,57.79 9.61,61.28 J1.3 | R14.1 37.55,55.56 24.53,55.56 22.94,53.97 9.61,53.97 J1.1
  Bottom 0.254: J1.2 9.61,57.47 9.61,53.97 J1.1
REF
  Bottom 0.305: JP5..5 81.04,10.38 80.08,11.35 80.08,12.15 81.04,13.11 JP5.5
RFU2
  Top 0.305: JP5..16 JP5.16
RO
  Top 0.254: 51.2,56.2 50.56,55.56 48.34,55.56 R3.2 | 51.2,56.2 51.2,57.47 R1.2 | IC11.15 80.73,57.15 69.3,57.15 68.98,56.83 60.09,56.83 58.82,55.56 51.84,55.56 51.2,56.2
SOUDIN
  Top 0.254: JP5.49 18.5,13.65 18.5,16.83 18.81,17.14 19.45,17.14 19.45,21.91 C14.+
  Bottom 0.305: JP5..49 25.16,10.38 24.2,11.35 24.2,12.15 25.16,13.11 JP5.49
SW
  Top 0.305: JP5..46 30.25,11.49 | 30.25,11.49 JP5.46 | JP5..44 JP5.44 30.5,11.75 30.25,11.49
V+  (via drill 0.35)
  Top 0.254: v32.47,57.47 R11.2 | v30.25,41.28 28.97,40 C12.+ 28.97,39.69 30.56,39.69 30.56,35.88 30.25,35.56 25.16,35.56 AMS1.3 | JP5.48 28.97,13.02 v28.97,18.41
  Top 0.305: JP5..48 JP5.48
  Bottom 0.254: v32.47,57.47 30.25,55.25 v30.25,41.28 30.88,40.64 30.88,20.32 v28.97,18.41
V-
  Top 0.254: JP5.50 12.47,11.75 12.47,46.99 14.05,48.58 30.88,48.58 30.88,53.66 R12.2
  Top 0.305: JP5..50 JP5.50
VCC  (via drill 0.35)
  Top 0.254: 34.69,34.93 36.91,37.15 IC1.28 37.86,44.45 C13.1 | 34.69,34.93 C11.1 34.69,34.93 | JP5.47 26.75,14.61 21.04,14.61 20.08,15.56 C5.+ | 34.69,34.93 37.23,32.39 37.23,30.16 36.28,30.16 30.88,24.77 30.88,13.65 JP5.45 | 67.71,59.69 67.71,60.01 IC3.14 | 67.71,59.69 67.71,58.74 IC3.13 | C10.1 55.96,62.55 55.64,62.23 55.64,60.01 IC3.1 IC3.14 | 82.31,28.89 86.12,28.89 U$3.1 | C13.1 78.5,45.72 85.17,45.72 85.81,46.36 85.81,48.26 80.73,48.26 IC2.14 | v78.19,56.2 IC3.11 | 82.31,28.89 82,29.21 v80.73,29.21 | 82.31,28.89 U$1.1 | 67.71,59.69 78.19,59.69 v78.5,59.37 | 67.71,59.69 IC3.14 | C13.1
  Bottom 0.254: 80.73,48.26 80.73,53.66 v78.19,56.2 78.19,59.06 v78.5,59.37 | IC2.14 80.73,48.26 | 80.73,48.26 v80.73,29.21
  Bottom 0.305: JP5..45 30.25,10.38 29.28,11.35 29.28,12.15 30.25,13.11 30.25,13.53 | 30.25,13.53 JP5.45 | JP5..47 27.7,10.38 26.74,11.35 26.74,12.15 27.7,13.11 JP5.47 30.12,13.65 30.25,13.53

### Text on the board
tPlace: RD/Oe/CS1 | GND/A14/VCC | GND/A15/VCC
